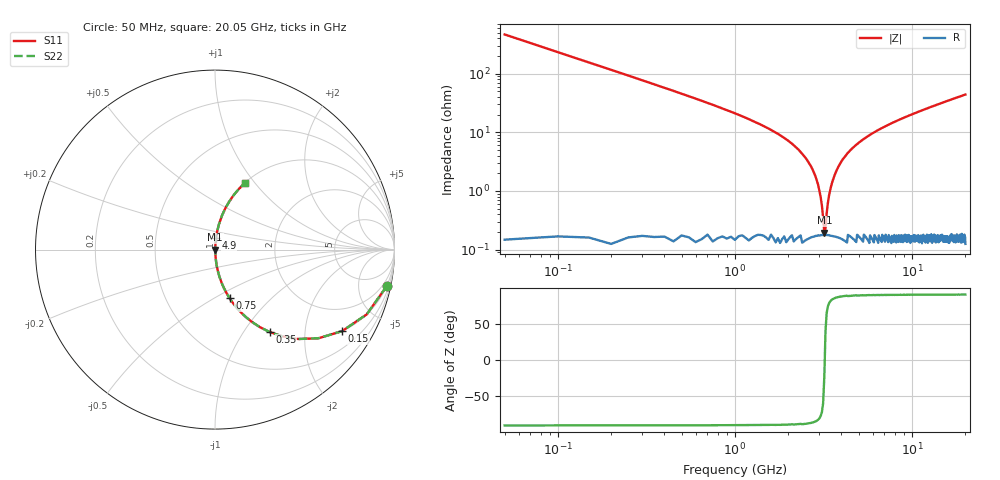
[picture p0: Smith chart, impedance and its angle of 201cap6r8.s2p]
! AVX Thin Film Operation		Date: May 2007
! Description: Accu-P® Series, Thin Film, SMD, RF Capacitor
! Part Number: 0201ZK6R8ABS
! 50 MHz  -  20.05 GHz
! Serial Measurements
# MHZ S MA R 50
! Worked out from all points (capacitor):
!   401 points, 50 MHz to 20.05 GHz, reference 50 ohm
!   read as one part in series: C = 6.8 pF near 150 MHz
!   lowest |Z| = 193 mohm at 3.2 GHz (marker M1)
!   series resonance near 3.217 GHz, so ESL is about 360 pH
!   S11 on the Smith chart (normalised r, x): 50 MHz: 1.00, -9.36; 150 MHz: 1.00, -3.11; 350 MHz: 1.00, -1.32; 750 MHz: 1.00, -0.59; 4.9 GHz: 1.00, +0.13; 20.05 GHz: 1.00, +0.88
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50  0.978 -12.1  0.209 77.9  0.209 77.9  0.978 -12.1
150  0.841 -32.7  0.54 57.2  0.54 57.2  0.841 -32.7
250  0.681 -47.0  0.731 42.9  0.731 42.9  0.681 -47.0
350  0.551 -56.5  0.833 33.4  0.833 33.4  0.551 -56.5
500  0.415 -65.3  0.908 24.5  0.908 24.5  0.415 -65.3
750  0.283 -73.3  0.958 16.4  0.958 16.4  0.283 -73.3
1450  0.127 -82.0  0.99 7.3  0.99 7.3  0.127 -82.0
2150  0.06 -85.1  0.997 3.4  0.997 3.4  0.06 -85.1
2600  0.031 -85.4  0.998 1.8  0.998 1.8  0.031 -85.4
2950  0.013 -82.3  0.998 0.7  0.998 0.7  0.013 -82.3
3150  0.003417 -62.9  0.998 0.2  0.998 0.2  0.003417 -62.9
3200  0.001723 -26.0  0.998 0.0  0.998 0.0  0.001723 -26.0
3300  0.004023 67.2  0.998 -0.2  0.998 -0.2  0.004023 67.2
3400  0.008202 78.7  0.998 -0.5  0.998 -0.5  0.008202 78.7
3600  0.016 83.7  0.998 -0.9  0.998 -0.9  0.016 83.7
3900  0.028 85.2  0.998 -1.6  0.998 -1.6  0.028 85.2
4900  0.063 85.0  0.996 -3.6  0.996 -3.6  0.063 85.0
6750  0.117 82.5  0.992 -6.7  0.992 -6.7  0.117 82.5
10050  0.2 78.0  0.978 -11.5  0.978 -11.5  0.2 78.0
13400  0.274 73.8  0.96 -15.9  0.96 -15.9  0.274 73.8
16750  0.342 69.7  0.938 -20.0  0.938 -20.0  0.342 69.7
20050  0.404 66.0  0.914 -23.8  0.914 -23.8  0.404 66.0
